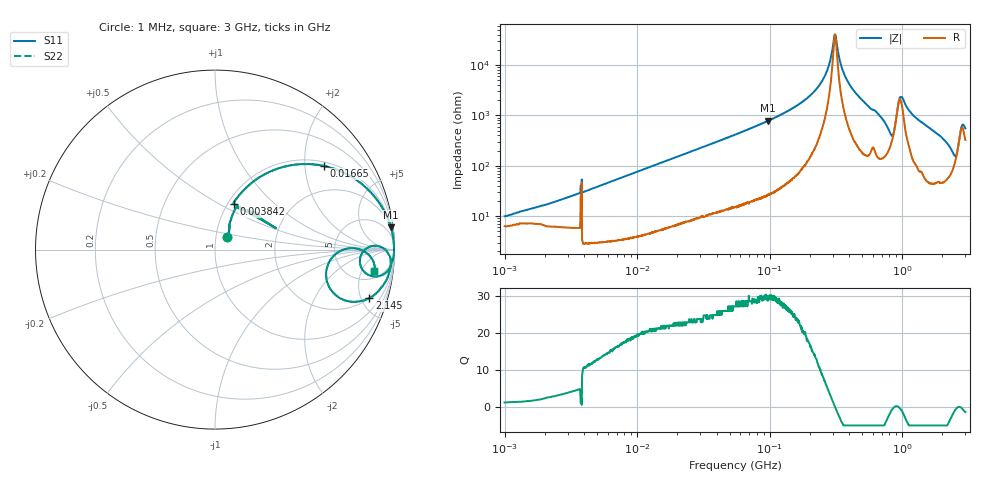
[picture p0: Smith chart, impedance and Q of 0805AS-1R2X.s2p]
!s-Parameter Generated by FASTRON Sdn. Bhd.
!FASTRON P/N : 0805AS-1R2X
!Keysight Technologies: E4991B_MY54100416_A.01.15
!Date: Mon Jun 15 12:56:44 2026
!Version  :Rev01  Mon Jun 15 12:56:44 2026
!Data & Calibration Information:
!Freq  S11  S21  S12  S22
!PortZ  Port1:50+j0  Port2:50+j0
!When reading reference impedance value at option line is always used.
! Remarks : This data is being provided solely for informational purposes.
# Hz S dB R 50
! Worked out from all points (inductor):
!   1601 points, 1 MHz to 3 GHz, reference 50 ohm
!   read as one part in series: L = 1.22 uH near 2.425 MHz
!   highest Q = 29.8 at 97.38 MHz (marker M1), where L = 1.28 uH
!   self-resonance near 310.9 MHz
!   S11 on the Smith chart (normalised r, x): 1 MHz: 1.13, +0.15; 3.842 MHz: 1.07, +0.59; 16.65 MHz: 1.11, +2.51; 2.145 GHz: 2.04, -5.84; 3 GHz: 8, -9
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1000000  -20.60 46.3  -0.56 -4.1  -0.56 -4.1  -20.60 46.3
3804036  -10.90 50.0  -1.45 -14.9  -1.45 -14.9  -10.90 50.0
3842298  -11.20 67.6  -0.63 -15.8  -0.63 -15.8  -11.20 67.6
6530558  -7.23 60.6  -1.18 -25.7  -1.18 -25.7  -7.23 60.6
1.447069e7  -2.83 41.2  -3.62 -46.1  -3.62 -46.1  -2.83 41.2
1.664711e7  -2.32 37.5  -4.31 -49.9  -4.31 -49.9  -2.32 37.5
5.504702e7  -0.32 13.4  -12.70 -74.5  -12.70 -74.5  -0.32 13.4
9.738201e7  -0.11 7.3  -18.00 -80.8  -18.00 -80.8  -0.11 7.3
2.083556e8  -0.03 2.1  -28.60 -84.1  -28.60 -84.1  -0.03 2.1
2.649225e8  -0.02 0.9  -36.40 -80.1  -36.40 -80.1  -0.02 0.9
3.124888e8  -0.02 -0.0  -52.00 4.5  -52.00 4.5  -0.02 -0.0
3.523638e8  -0.02 -0.7  -38.50 76.0  -38.50 76.0  -0.02 -0.7
4.013235e8  -0.03 -1.4  -32.20 81.3  -32.20 81.3  -0.03 -1.4
7.925923e8  -0.76 -9.4  -15.00 57.4  -15.00 57.4  -0.76 -9.4
8.543737e8  -1.83 -3.6  -14.00 14.8  -14.00 14.8  -1.83 -3.6
9.443041e8  -0.44 -0.1  -26.20 2.8  -26.20 2.8  -0.44 -0.1
9.878038e8  -0.29 -1.6  -27.50 39.1  -27.50 39.1  -0.29 -1.6
1.237271e9  -0.15 -5.9  -19.70 77.2  -19.70 77.2  -0.15 -5.9
2.145442e9  -0.90 -17.4  -10.30 62.6  -10.30 62.6  -0.90 -17.4
2.505452e9  -3.74 -16.1  -7.61 25.6  -7.61 25.6  -3.74 -16.1
2.811057e9  -1.29 -2.3  -16.90 13.7  -16.90 13.7  -1.29 -2.3
3e9  -0.96 -7.5  -15.80 46.3  -15.80 46.3  -0.96 -7.5
